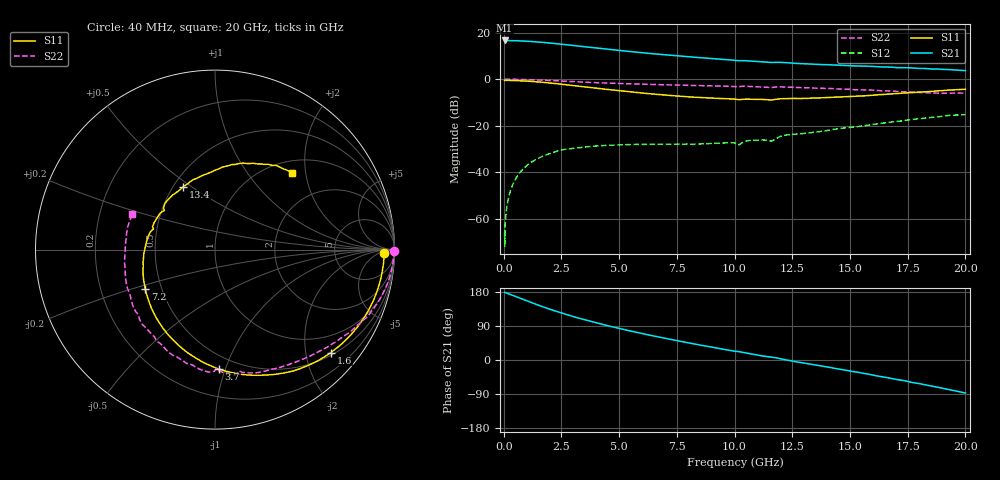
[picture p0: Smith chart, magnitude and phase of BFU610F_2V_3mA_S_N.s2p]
! Filename:  P:\Prog\Test\Noise\ATS_data\Testdata_Net\SplitFiles\BFU610_2W_A5_HighFreq_2V_3mA_D.s2p
! Date/Time: Wed 10/Aug/2011 16:55:54
! BFU610_2W_A5_HighFreq_2V_1mA_10mA_Bias3_R.s2p
! MDIF S-parameter v. bias file
! BFU610_2W_A5_HighFreq_2V_1mA_10mA
! Date/time Mon Aug 08 14:20:39 2011
! VAR V_out= 2.0002
! VAR I_out= 2.9900
! VAR V_in= 0.8821
! VAR I_in= 0.0232
! Device data file deembeded for feedlines and parallel
! Original file: \SplitFiles\BFU610_2W_A5_HighFreq_2V_3mA_R.s2p
! Feed-files: PR003V01_101208_Feed1.s2p, PR003V01_101208_Feed2.s2p
! Parallel-file: PR003V01_101208_Par.s2p
# MHz S MA R 50
!  Freq-MHz  S11-mag  S11-arg  S21-mag  S21-arg  S12-mag  S12-arg  S22-mag  S22-arg
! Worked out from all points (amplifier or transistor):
!   167 points, 40 MHz to 20 GHz, reference 50 ohm
!   highest |S21| = 16.7 dB at 40 MHz (marker M1)
!   |S21| within 3 dB of that: start of sweep to 3.799 GHz
!   unconditionally stable (mu >= 1): 5.924 GHz to 18.24 GHz
!   at 550 MHz: K = 0.03, MSG = 29.5 dB, |S12| = -42.4 dB
!   at 4.2 GHz: K = 0.66, MSG = 20.9 dB, |S12| = -28.6 dB
!   at 20 GHz: K = 0.87, MSG = 9.4 dB, |S12| = -15.2 dB
!   lowest NFmin = 1.03 dB at 400 MHz
!   S11 on the Smith chart (normalised r, x): 40 MHz: 31, -10; 1.6 GHz: 0.56, -2.52; 3.7 GHz: 0.40, -0.95; 7.2 GHz: 0.40, -0.22; 13.4 GHz: 0.56, +0.46; 20 GHz: 1.24, +1.68
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40  0.9426 -1.1  6.804 178.8  0.0005028 87.2  0.9947 -0.3
50  0.9353 -1.6  6.777 178.9  0.0002552 95.8  0.995 -0.5
60  0.9423 -1.3  6.796 178.0  0.0007032 104.2  0.9958 -0.6
140  0.9422 -3.7  6.773 176.5  0.001832 91.1  0.9959 -1.6
460  0.935 -12.3  6.734 168.8  0.006357 85.5  0.9925 -5.4
950  0.911 -25.3  6.586 157.1  0.01314 75.9  0.9797 -10.9
1600  0.8641 -41.6  6.232 142.6  0.02101 64.8  0.9538 -17.9
2050  0.8226 -52.5  5.966 133.0  0.02542 58.2  0.9335 -22.4
2500  0.7775 -62.9  5.654 124.0  0.02968 51.9  0.908 -26.6
3400  0.6931 -81.9  5.053 108.0  0.03429 41.6  0.8657 -33.9
3700  0.6665 -88.0  4.875 103.1  0.03553 38.9  0.8523 -36.1
4400  0.6079 -101.5  4.466 92.0  0.03751 33.5  0.8276 -41.1
5200  0.5507 -116.1  4.056 80.6  0.03891 29.1  0.8014 -46.6
6800  0.4626 -143.9  3.404 59.6  0.03979 24.2  0.7614 -57.2
7200  0.4464 -150.8  3.272 54.8  0.03991 23.9  0.7527 -59.9
8600  0.401 -173.6  2.883 38.5  0.04055 25.8  0.729 -69.1
10200  0.3612 161.6  2.495 22.0  0.03873 30.5  0.6926 -78.5
12000  0.379 137.6  2.296 3.1  0.05927 40.9  0.6832 -92.8
13400  0.393 117.1  2.097 -12.0  0.07173 32.7  0.6436 -106.2
16800  0.4832 78.6  1.815 -48.8  0.1197 16.9  0.5544 -145.6
18800  0.5599 58.1  1.654 -71.8  0.1553 -0.1  0.5004 -178.7
20000  0.6062 45.0  1.527 -87.0  0.1735 -13.4  0.5009 156.6
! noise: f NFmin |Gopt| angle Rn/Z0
400  1.03  0.6498  3.2  0.5372
700  1.056  0.6348  6.738  0.5357
1150  1.095  0.6147  11.91  0.5318
1600  1.135  0.597  16.9  0.5259
2050  1.177  0.5807  21.71  0.5182
2600  1.23  0.5619  27.37  0.5064
3500  1.32  0.5314  36.25  0.4818
4400  1.415  0.4996  44.96  0.4509
5600  1.55  0.4547  57.13  0.4013
8000  1.845  0.3808  87.88  0.2779
